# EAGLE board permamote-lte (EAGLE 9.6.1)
REV: C
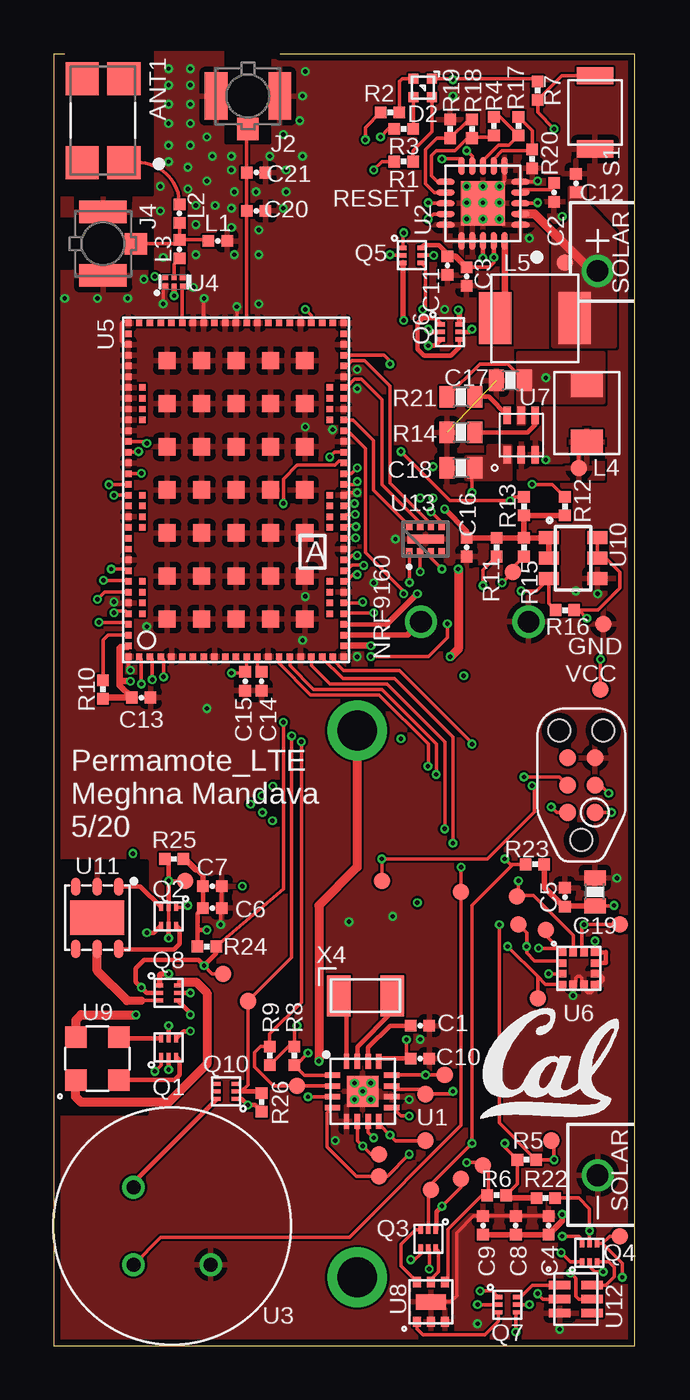
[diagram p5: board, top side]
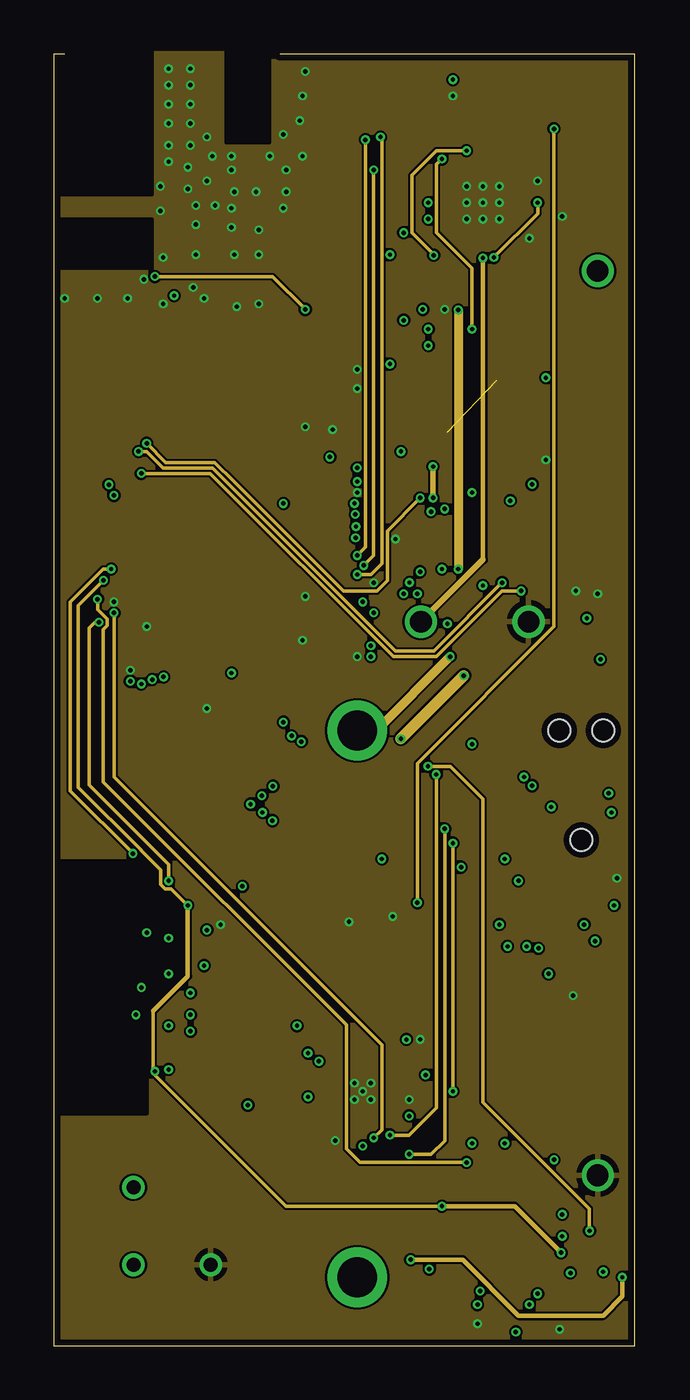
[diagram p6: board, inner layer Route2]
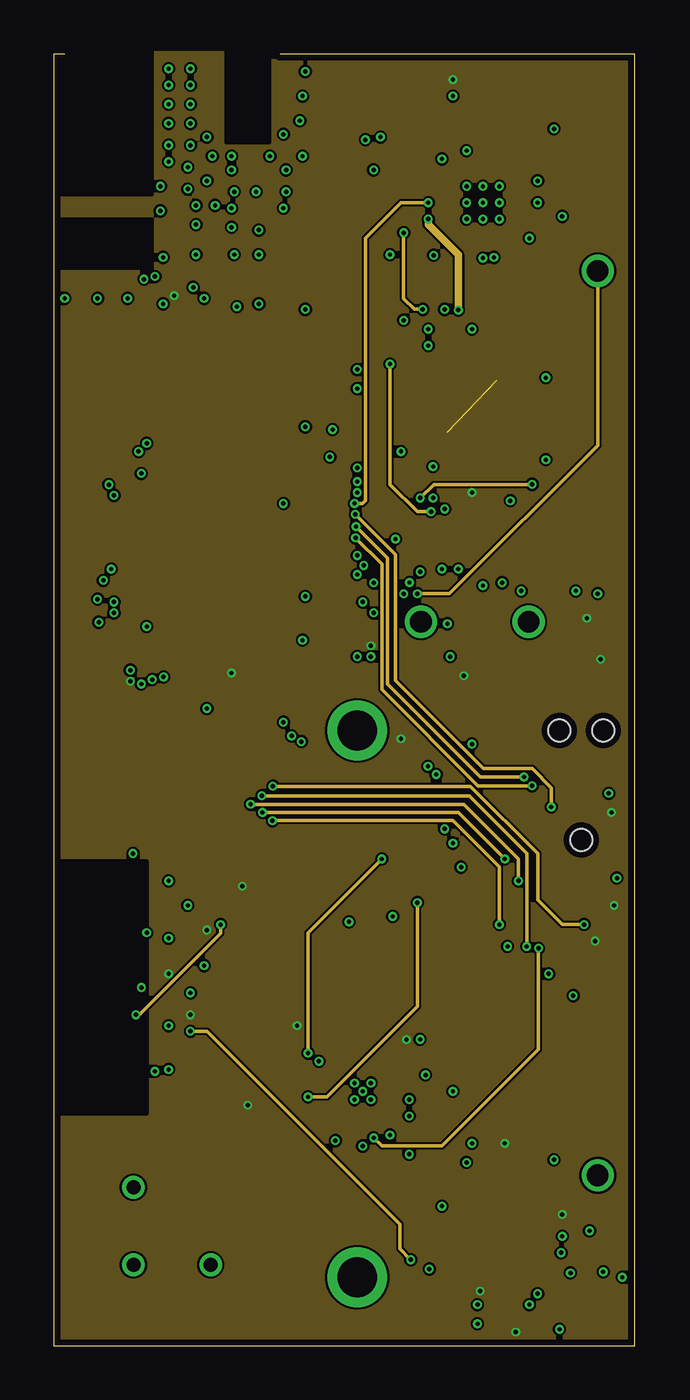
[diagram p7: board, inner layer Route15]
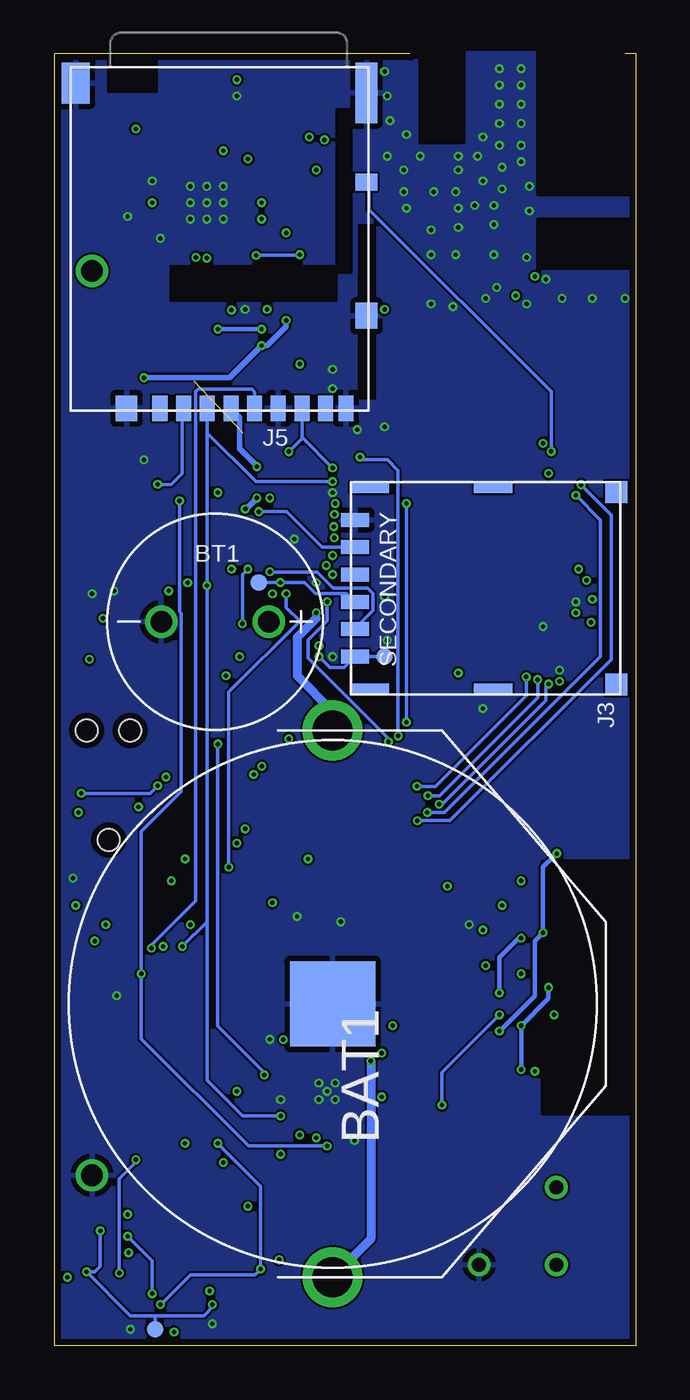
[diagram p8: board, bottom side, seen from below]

Size 27 x 60 mm. Coordinates in mm from the lower left corner, seen from the top.
Outline: 0.5,60 0,60 0,0 27,0 27,60 10.5,60
Copper layers (1+2*15+16): Top 0.0178mm / dielectric 59mil / Route2 0.0356mm / dielectric 0.1499mm / Route15 0.0356mm / dielectric 0.2007mm / Bottom 0.0178mm
Design rules "quickturn_co_kr_1oz_4lyr *": minimum track width 4mil, minimum drill 8mil, track to track 4mil, track to pad 4mil, pad to pad 4mil, via to via 4mil, smd to smd 4mil, copper to edge 12mil, drill to drill 12mil, minimum pad ring 8mil, minimum via ring 4mil, stop-mask expansion 3mil, vias tented up to drill 50mil, thermal gap 10mil
tKeepout: area 24.9,18 to 25.4,18
tRestrict: area 24.4,16.5 to 24.4,17; area 24.9,16.5 to 24.9,17; area 24.9,17 to 25.4,17; area 17.8,0.9 to 17.9,1.5

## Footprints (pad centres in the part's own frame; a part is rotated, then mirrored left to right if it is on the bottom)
ANT_1462350001 = smd 1.54 x 1.54: 1 -1.95,-0.97; 2 1.95,-0.97; 3 1.95,0.97; 4 -1.95,0.97
2477THMCOINCLIP = drill 1.854: 1 -12.7,0; 2 12.7,0 | smd 3.962 x 3.962: GND 0,0
1020 = drill 1: + -2.5,0; - 2.5,0
0402_CAP = smd 0.536 x 0.546: 1 -0.433,0; 2 0.433,0
0603_CAP = smd 0.7 x 1: 1 -0.65,0; 2 0.65,0
SOLAR_HOLES = drill 1: + 0,0; - 42,0
1MM_SQ_4PAD = smd 0.457 x 0.457: 1 0.432,0.432; 2 0.432,-0.432; 3 -0.432,-0.432; 4 -0.432,0.432
TC2030-IDC-NL = smd 0.787 x 0.787: 1 -1.27,-0.635; 2 -1.27,0.635; 3 0,-0.635; 4 0,0.635; 5 1.27,-0.635; 6 1.27,0.635 | hole 1.016: -2.54,0; 2.54,1.016; 2.54,-1.016
U.FL_SMT = smd 1.05 x 2.2: GND1 -1.475,0; GND2 1.475,0 | smd 1 x 1.05: SIG 0,-1.525
WURTH_NANO_SIM = smd 0.65 x 1.3: C1 1.905,6.07; C2 -0.635,6.07; C3 -1.905,6.07; C5 3.175,6.07; C6 0.635,6.07; C7 -3.175,6.07 | smd 1.03 x 1: P$8 -4.465,-6.07; P$9 4.465,-6.07 | smd 0.48 x 1.8: P$10 -4.66,-0.35; P$11 4.66,-0.35; P$12 -4.66,5.4; P$13 4.66,5.4
DM3AT-SF-PEJM5 = smd 0.7 x 1.2: 1 3.2,-0.1; 2 2.1,-0.1; 3 1,-0.1; 4 -0.1,-0.1; 5 -1.2,-0.1; 6 -2.3,-0.1; 7 -3.4,-0.1; 8 -4.5,-0.1; B -5.45,-0.1 | smd 1 x 0.8: A -6.4,-10.6 | smd 1 x 1.2: MOUNT0 4.75,-0.1; MOUNT1 -6.4,-4.4 | smd 1 x 2.8: MOUNT2 -6.4,-14.75 | smd 1.3 x 1.9: MOUNT3 7.1,-15.2
IHL-1212BZ-11 = smd 1.2 x 1.5: P$1 -1.35,0; P$2 1.35,0
74437324220 = smd 1.5 x 2.4: P$1 1.85,0; P$2 -1.85,0
XDFN-6 = smd 0.35 x 0.2: 1 -0.425,0.35; 2 -0.425,0; 3 -0.425,-0.35; 4 0.425,-0.35; 5 0.425,0; 6 0.425,0.35
0402_RES = smd 0.536 x 0.546: 1 -0.433,0; 2 0.433,0
0603-RES = smd 0.7 x 1: 1 -0.65,0; 2 0.65,0
B3U-1000P = smd 0.8 x 1.7: 1 -1.7,0; 2 1.7,0
PAD.03X.03 = smd 0.762 x 0.762: P$1 0,0
QFN-16-3MM = smd 0.7 x 0.25: 1 -1.4,0.75; 2 -1.4,0.25; 3 -1.4,-0.25; 4 -1.4,-0.75; 9 1.35,-0.75; 10 1.35,-0.25; 11 1.35,0.25; 12 1.35,0.75 | smd 0.25 x 0.7: 5 -0.75,-1.4; 6 -0.25,-1.4; 7 0.25,-1.4; 8 0.75,-1.4; 13 0.75,1.4; 14 0.25,1.4; 15 -0.25,1.4; 16 -0.75,1.4 | smd 1.45 x 1.45: GND 0,0
S-PVQFN-N20-RGR = smd 0.28 x 0.85: 1 -1,-1.74; 2 -0.5,-1.74; 3 0,-1.74; 4 0.5,-1.74; 5 1,-1.74; 11 1,1.74; 12 0.5,1.74; 13 0,1.74; 14 -0.5,1.74; 15 -1,1.74 | smd 0.85 x 0.28: 6 1.74,-1; 7 1.74,-0.5; 8 1.74,0; 9 1.74,0.5; 10 1.74,1; 16 -1.74,1; 17 -1.74,0.5; 18 -1.74,0; 19 -1.74,-0.5; 20 -1.74,-1 | smd 2.05 x 2.05: PAD 0,0
AMN2 = drill 0.65: GND 1.796,-1.796; OUT -1.796,-1.796; VCC -1.796,1.796
LNA-TSLP-6-2-ORIG = smd 0.25 x 0.25: 1 -0.2,0.4; 2 -0.2,0; 3 -0.2,-0.4; 4 0.2,-0.4; 5 0.2,0; 6 0.2,0.4
NRF9160 = smd 0.3 x 0.3: ANT 15.75,4.75; AUX 15.75,6.25; COEX0 5.25,10.25; COEX1 5.75,10.25; COEX2 6.25,10.25; ENABLE 1.25,10.25; GND_SHIELD@1 0.25,10.25; GND_SHIELD@2 0.25,8.25; GND_SHIELD@3 0.25,6.25; GND_SHIELD@4 0.25,3.75; GND_SHIELD@5 0.25,2.25; GND_SHIELD@6 0.25,0.25; GND_SHIELD@7 3.25,0.25; GND_SHIELD@8 5.25,0.25; GND_SHIELD@9 7.75,0.25; GND_SHIELD@10 10.25,0.25; GND_SHIELD@11 11.75,0.25; GND_SHIELD@12 13.25,0.25; GND_SHIELD@13 14.75,0.25; GND_SHIELD@14 15.75,0.25; GND_SHIELD@15 15.75,2.25; GND_SHIELD@16 15.75,4.25; GND_SHIELD@17 15.75,5.25; GND_SHIELD@18 15.75,5.75; GND_SHIELD@19 15.75,6.75; GND_SHIELD@20 15.75,7.25; GND_SHIELD@21 15.75,10.25; GND_SHIELD@22 14.75,10.25; GND_SHIELD@23 14.25,10.25; GND_SHIELD@24 13.75,10.25; GND_SHIELD@25 13.25,10.25; GND_SHIELD@26 12.75,10.25; GND_SHIELD@27 12.25,10.25; GND_SHIELD@28 11.75,10.25; GND_SHIELD@29 11.25,10.25; GND_SHIELD@30 10.75,10.25; GND_SHIELD@31 9.25,10.25; GND_SHIELD@32 6.75,10.25; GND_SHIELD@33 4.75,10.25; GND_SHIELD@34 2.75,10.25; GPS 15.75,7.75; IO_SUPPLY 0.25,4.25; MAGPIO0 15.75,1.75; MAGPIO1 15.75,1.25; MAGPIO2 15.75,0.75; NC1 0.25,7.75; NC2 0.25,7.25; NC3 0.25,6.75; NC4 0.25,5.75; NC5 0.25,5.25; NC6 15.25,0.25; NC7 15.75,8.25; NC8 15.75,8.75; NC9 15.75,9.25; NC10 15.75,9.75; NC11 15.25,10.25; NC12 2.25,0.9; NC13 2.75,0.9; NC14 3.25,0.9; NC15 3.75,0.9; NC16 6.25,0.9; NC17 6.75,0.9; NC18 7.25,0.9; NC19 7.75,0.9; NC20 11.25,0.9; NC21 11.75,0.9; NC22 12.25,0.9; NC23 12.75,0.9; NC24 12.75,9.6; NC25 12.25,9.6; NC26 11.75,9.6; NC27 11.25,9.6; NC28 7.75,9.6; NC29 7.25,9.6; NC30 6.75,9.6; NC31 6.25,9.6; NC32 3.75,9.6; NC33 3.25,9.6; NC34 2.75,9.6; NC35 2.25,9.6; NRESET 5.75,0.25; P0.00 4.25,10.25; P0.01 3.75,10.25; P0.02 3.25,10.25; P0.03 2.25,10.25; P0.04 1.75,10.25; P0.05 0.25,9.75; P0.06 0.25,9.25; P0.07 0.25,8.75; P0.08 0.25,3.25; P0.09 0.25,2.75; P0.10 0.25,1.75; P0.11 0.25,1.25; P0.12 0.25,0.75; P0.13 1.25,0.25; P0.14 1.75,0.25; P0.15 2.25,0.25; P0.16 2.75,0.25; P0.17 3.75,0.25; P0.18 4.25,0.25; P0.19 4.75,0.25; P0.20 7.25,0.25; P0.21 8.25,0.25; P0.22 8.75,0.25; P0.23 9.25,0.25; P0.24 9.75,0.25; P0.25 10.75,0.25; P0.26 10.25,10.25; P0.27 9.75,10.25; P0.28 8.75,10.25; P0.29 8.25,10.25; P0.30 7.75,10.25; P0.31 7.25,10.25; SCLK 15.75,3.25; SDATA 15.75,3.75; SIM_1V8 14.25,0.25; SIM_CLK 12.75,0.25; SIM_DET 12.25,0.25; SIM_IO 13.75,0.25; SIM_RST 11.25,0.25; SWDCLK 6.25,0.25; SWDIO 6.75,0.25; VDD@1 0.75,0.25; VDD@2 0.75,10.25; VDD_GPIO 0.25,4.75; VIO 15.75,2.75 | smd 0.8 x 0.8: GND@1 2,8.45; GND@2 4,8.45; GND@3 6,8.45; GND@4 8,8.45; GND@5 10,8.45; GND@6 12,8.45; GND@7 14,8.45; GND@8 2,6.85; GND@9 4,6.85; GND@10 6,6.85; GND@11 8,6.85; GND@12 10,6.85; GND@13 12,6.85; GND@14 14,6.85; GND@15 2,5.25; GND@16 4,5.25; GND@17 6,5.25; GND@18 8,5.25; GND@19 10,5.25; GND@20 12,5.25; GND@21 14,5.25; GND@22 2,3.65; GND@23 4,3.65; GND@24 6,3.65; GND@25 8,3.65; GND@26 10,3.65; GND@27 12,3.65; GND@28 14,3.65; GND@29 2,2.05; GND@30 4,2.05; GND@31 6,2.05; GND@32 8,2.05; GND@33 10,2.05; GND@34 12,2.05; GND@35 14,2.05
LGA-12 = smd 0.375 x 0.35: 1 -0.75,0.75; 2 -0.75,0.25; 3 -0.75,-0.25; 4 -0.75,-0.75; 7 0.75,-0.75; 8 0.75,-0.25; 9 0.75,0.25; 10 0.75,0.75 | smd 0.35 x 0.375: 5 -0.25,-0.75; 6 0.25,-0.75; 11 0.25,0.75; 12 -0.25,0.75
UDFN-6-MAXIM = smd 0.8 x 0.35: 1 -0.915,0.65; 2 -0.915,0; 3 -0.915,-0.65; 4 0.915,-0.65; 5 0.915,0; 6 0.915,0.65
UDFN-6-EXPOSED = smd 0.48 x 0.36: 1 -0.925,0.65; 2 -0.925,0; 3 -0.925,-0.65; 4 0.925,-0.65; 5 0.925,0; 6 0.925,0.65 | smd 0.71 x 1.4: EP 0,0
4-SMD = smd 1 x 1: 1 -1,1; 2 -1,-1; 3 1,-1; 4 1,1
TSOT23-6 = smd 0.6 x 0.927: 1 -0.95,-1.126; 2 0,-1.126; 3 0.95,-1.126; 4 0.95,1.126; 5 0,1.126; 6 -0.95,1.126
DFN-6/3MM = smd 0.85 x 0.45: 1 -1.45,1; 2 -1.45,0; 3 -1.45,-1; 4 1.45,-1; 5 1.45,0; 6 1.45,1 | smd 1.6 x 2.5: P$1 0,0
FN-6 = smd 1 x 0.4: 1 -0.75,0.65; 2 -0.75,0; 3 -0.75,-0.65; 4 0.75,-0.65; 5 0.75,0; 6 0.75,0.65
DPV8_1P7X0P4 = smd 0.38 x 0.3: 1 -0.61,0.75; 2 -0.61,0.25; 3 -0.61,-0.25; 4 -0.61,-0.75; 5 0.61,-0.75; 6 0.61,-0.25; 7 0.61,0.25; 8 0.61,0.75 | smd 0.4 x 1.7: 9 0,0
2-SMD = smd 1.092 x 1.905: 1 -1.245,0; 2 1.245,0

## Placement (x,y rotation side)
ANT1  1462350001  [ANT_1462350001]  2.29,56.9 90 top
BAT1  2477THMCOINCELLCLIP  [2477THMCOINCLIP]  14.1,15.88 90 bottom
BT1  LTOHTC1020  [1020]  19.56,33.62 180 bottom
C1  47pF  [0402_CAP]  17.02,14.86 0 top
C2  10nF  [0402_CAP]  23.24,53.56 270 top
C3  10nF  [0402_CAP]  19.18,49.66 270 top
C4  0.1uF  [0402_CAP]  22.99,5.59 90 top
C5  0.1uF  [0402_CAP]  23.75,20.83 90 top
C6  0.1uF  [0402_CAP]  7.37,20.32 0 top
C7  0.1uF  [0402_CAP]  7.37,21.34 0 top
C8  1uF  [0402_CAP]  21.46,5.59 90 top
C9  1uF  [0402_CAP]  19.94,5.59 90 top
C10  1uF  [0402_CAP]  17.02,13.34 0 top
C11  4.7uF  [0402_CAP]  18.29,50.16 270 top
C12  4.7uF  [0402_CAP]  24.26,53.99 90 top
C13  4.7uF  [0402_CAP]  4.06,30.1 0 top
C14  4.7uF  [0402_CAP]  9.65,30.86 270 top
C15  4.7uF  [0402_CAP]  8.89,30.86 270 top
C16  4.7uF  [0402_CAP]  19.18,37.08 270 top
C17  10uF  [0603_CAP]  21.21,44.83 180 top
C18  10uF  [0603_CAP]  18.92,40.77 180 top
C19  10uF  [0603_CAP]  25.15,21.08 90 top
C20  DNP  [0402_CAP]  9.4,52.7 180 top
C21  DNP  [0402_CAP]  9.4,54.48 180 top
D1  SOLARCELLHOLES  [SOLAR_HOLES]  25.27,49.91 270 top
D2  SML-LX0404SIUPGUSB  [1MM_SQ_4PAD]  17.14,58.42 0 top
J1  TC2030-JLINK-NL  [TC2030-IDC-NL]  24.51,26.04 90 top
J2  U.FL-R-SMT  [U.FL_SMT]  9.02,58.04 0 top
J3  NANO_SIM  [WURTH_NANO_SIM]  6.99,35.18 90 bottom
J4  U.FL-R-SMT  [U.FL_SMT]  2.29,51.18 90 top
J5  DM3AT-SF-PEJM5  [DM3AT-SF-PEJM5]  18.92,43.43 180 bottom
L1  1.8nH  [0402_CAP]  7.62,51.31 180 top
L2  5.1nH  [0402_CAP]  5.84,52.58 90 top
L3  7.5nH  [0402_CAP]  5.84,50.93 90 top
L4  1uH  [IHL-1212BZ-11]  24.77,43.31 270 top
L5  22uH  [74437324220]  22.35,47.72 180 top
Q1  PMDXB950UPEL  [XDFN-6]  5.33,13.84 90 top
Q2  PMDXB950UPEL  [XDFN-6]  5.33,19.94 270 top
Q3  PMDXB950UPEL  [XDFN-6]  17.4,4.95 270 top
Q4  PMDXB950UPEL  [XDFN-6]  24.89,4.32 90 top
Q5  PMDXB950UPEL  [XDFN-6]  16.64,50.64 0 top
Q6  PMDXB950UPEL  [XDFN-6]  18.41,47.09 0 top
Q7  PMDXB950UPEL  [XDFN-6]  21.08,1.91 0 top
Q8  PMDXB950UPEL  [XDFN-6]  5.33,16.38 0 top
Q10  PMDXB950UPEL  [XDFN-6]  8,11.81 180 top
R1  470  [0402_RES]  16.26,54.99 180 top
R2  470  [0402_RES]  15.62,57.28 180 top
R3  470  [0402_RES]  16.26,56.52 180 top
R4  6.04k  [0402_RES]  20.45,56.64 90 top
R5  10k  [0402_RES]  21.97,8.64 180 top
R6  10k  [0402_RES]  20.57,6.99 0 top
R7  10k  [0402_RES]  22.48,58.29 90 top
R8  10k  [0402_RES]  11.18,13.46 90 top
R9  10k  [0402_RES]  10.03,13.46 270 top
R10  10k  [0402_RES]  2.29,30.48 90 top
R11  10k  [0402_RES]  20.57,37.08 90 top
R12  10k  [0402_RES]  23.75,38.99 270 top
R13  10k  [0402_RES]  21.84,38.99 270 top
R14  80.6k  [0603-RES]  18.92,42.42 0 top
R15  100k  [0402_RES]  21.84,37.08 90 top
R16  100k  [0402_RES]  23.75,34.16 0 top
R17  3.9M  [0402_RES]  21.59,56.64 270 top
R18  6.2M  [0402_RES]  19.43,56.52 270 top
R19  6.8M  [0402_RES]  18.41,56.52 270 top
R20  9.1M  [0402_RES]  22.23,55.12 90 top
R21  33M  [0603-RES]  18.92,44.07 180 top
R22  100M  [0402_RES]  22.86,6.86 180 top
R23  100M  [0402_RES]  22.35,22.35 0 top
R24  100M  [0402_RES]  7.11,18.54 180 top
R25  100M  [0402_RES]  5.59,22.61 0 top
R26  100M  [0402_RES]  9.65,11.3 270 top
S1  B3U-1000P  [B3U-1000P]  25.15,57.28 90 top
TP1  TEST-POINT  [PAD.03X.03]  26.29,5.08 0 top
TP2  TEST-POINT  [PAD.03X.03]  18.92,7.75 0 top
TP3  TEST-POINT  [PAD.03X.03]  22.86,19.3 270 top
TP4  TEST-POINT  [PAD.03X.03]  15.11,8.89 0 top
TP5  TEST-POINT  [PAD.03X.03]  22.48,16.13 90 top
TP6  TEST-POINT  [PAD.03X.03]  18.16,12.57 0 top
TP7  TEST-POINT  [PAD.03X.03]  21.59,19.56 90 top
TP8  TEST-POINT  [PAD.03X.03]  7.87,17.27 0 top
TP9  TEST-POINT  [PAD.03X.03]  22.35,0.76 0 bottom
TP10  TEST-POINT  [PAD.03X.03]  17.53,7.24 0 top
TP11  TEST-POINT  [PAD.03X.03]  9.02,16 0 top
TP12  TEST-POINT  [PAD.03X.03]  6.1,21.59 0 top
TP13  TEST-POINT  [PAD.03X.03]  17.27,11.68 90 top
TP14  TEST-POINT  [PAD.03X.03]  15.11,7.87 0 top
TP15  TEST-POINT  [PAD.03X.03]  17.27,9.53 0 top
TP16  TEST-POINT  [PAD.03X.03]  11.3,12.06 0 top
TP17  TEST-POINT  [PAD.03X.03]  15.24,21.59 0 top
TP18  TEST-POINT  [PAD.03X.03]  21.51,20.87 0 top
TP19  TEST-POINT  [PAD.03X.03]  26.29,19.56 270 top
TP20  TEST-POINT  [PAD.03X.03]  23.11,9.53 0 top
TP21  TEST-POINT  [PAD.03X.03]  19.94,8.38 0 top
TP22  TEST-POINT  [PAD.03X.03]  18.92,21.08 90 top
TP23  TEST-POINT  [PAD.03X.03]  23.75,50.29 0 top
TP25  TEST-POINT  [PAD.03X.03]  24.38,40.77 0 top
TP26  TEST-POINT  [PAD.03X.03]  25.4,30.48 0 top
TP27  TEST-POINT  [PAD.03X.03]  25.53,33.53 0 top
TP30  TEST-POINT  [PAD.03X.03]  17.53,35.43 0 bottom
TP31  TEST-POINT  [PAD.03X.03]  11.68,32 270 bottom
TP32  TEST-POINT  [PAD.03X.03]  21.34,35.94 0 top
U1  AB1815-T3  [QFN-16-3MM]  14.35,11.81 0 top
U2  BQ25505  [S-PVQFN-N20-RGR]  19.94,53.05 90 top
U3  EKMB1101111  [AMN2]  5.5,5.56 0 top
U4  BGA725L6  [LNA-TSLP-6-2-ORIG]  5.59,49.4 90 top
U5  NRF9160  [NRF9160]  13.72,31.75 90 top
U6  LIS2DW12  [LGA-12]  24.38,17.53 0 top
U7  MAX17222  [UDFN-6-MAXIM]  21.72,42.29 90 top
U8  MAX44009  [UDFN-6-EXPOSED]  17.53,2.03 90 top
U9  MS5637-02BA03  [4-SMD]  2.03,13.34 90 top
U10  SIP32510  [TSOT23-6]  24.13,36.58 270 top
U11  SI7021-A20-GM1  [DFN-6/3MM]  2.02,19.88 270 top
U12  TCS34725  [FN-6]  24.26,2.16 0 top
U13  TPD3F303DPVR  [DPV8_1P7X0P4]  17.27,37.47 90 top
U$2  [UCB_CAL_200MIL]  19.81,10.54 0 top
X4  ABS07-32.768KHZ-7-T  [2-SMD]  14.48,16.26 0 top

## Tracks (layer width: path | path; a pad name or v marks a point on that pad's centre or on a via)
!CLR_EN  (via drill 0.2)
  Top 0.152: Q7.2 v19.68,1.91 | v25.53,3.43 25.15,3.43 24.89,3.68 Q4.2 | Q4.5 v24.89,5.33 24.89,6.35 24.38,6.86 R22.1 | U5.P0.08 10.47,31.7 11.94,30.23 15.11,30.23 17.4,27.94 17.4,26.92 v17.38,26.91
  Route2 0.152: v17.38,26.91 18.43,26.91 19.94,25.4 19.94,11.3 24.89,6.35 v24.89,5.33
  Bottom 0.152: v19.68,1.91 19.62,1.84 20.07,1.4 22.35,1.4 | v24.89,5.33 24.89,3.68 25.15,3.43 v25.53,3.43 23.5,1.4 22.35,1.4 | 22.35,1.4 TP9.P$1
!CLR_INT  (via drill 0.2)
  Top 0.152: U12.5 24.38,2.16 24.26,2.29 24.26,3.12 v24,3.38 | U5.P0.29 v2.56,40 v2.56,39.99 | TP20.P$1 23.24,9.4 v23.24,8.64 R5.1 20.7,10.34 v20.7,19.56
  Route15 0.152: v20.7,19.56 20.7,22.23 18.54,24.38 v10.16,24.38
  Bottom 0.152: v23.24,8.64 23.24,8.51 24,7.75 v24,3.38 | v2.56,39.99 1.14,38.58 1.14,31.88 8.64,24.38 v10.16,24.38
!HUM_EN  (via drill 0.2)
  Top 0.152: v2.09,33.59 3.37,33.59 U5.P0.04 | TP12.P$1 v5.33,21.59 | Q2.2 Q2.5
  Top 0.203: Q2.5 v5.33,18.92 | Q8.5 v6.35,16.38 | Q2.2 v5.33,21.59 5.33,22.43 R25.1
  Route2 0.152: v2.09,33.59 1.91,33.59 1.65,33.34 1.65,26.04 5.33,22.35 v5.33,21.59
  Bottom 0.203: v5.33,18.92 5.33,19.05 6.35,18.03 v6.35,16.38
!LT_EN  (via drill 0.2)
  Top 0.152: Q3.5 17.44,4.48 v17.44,3.56 | Q7.5 v22.1,1.91 | Q3.2 17.4,7.11 TP10.P$1 17.53,7.49 v19.43,9.4 19.43,20.45 21.34,22.35 | R23.1 21.34,22.35 | 21.34,22.35 21.21,22.35 v20.95,22.61 | U5.P0.30 v2.79,39.5
  Route15 0.152: v20.95,22.61 18.8,24.77 v9.7,24.77
  Bottom 0.152: v19.43,9.4 17.44,7.41 v17.44,3.56 17.7,3.3 20.7,3.3 v22.1,1.91 | v2.79,39.5 1.65,38.35 1.65,32 8.89,24.77 v9.7,24.77
!LT_INT  (via drill 0.2)
  Top 0.152: U8.4 18.3,3.08 18.3,5.4 19.89,6.99 R6.1 20.19,7.04 20.19,8.13 TP21.P$1 19.81,8.51 v19.18,8.51 | U5.P0.02 2.36,35 v2.03,34.67
  Route2 0.152: v2.03,34.67 2.03,34.19 2.47,33.75 2.47,33.44 2.29,33.25 2.29,26.19 13.59,14.89 13.59,9.14 14.22,8.51 v19.18,8.51
!PIR_EN  (via drill 0.2)
  Top 0.152: U5.P0.24 13.05,41.5 v12.83,41.27 | v11.05,28.32 11.05,18.03 TP11.P$1 9.02,12.12 8.71,11.81 Q10.2
  Top 0.203: Q10.2 9.58,11.81 R26.1
  Bottom 0.152: v11.05,28.32 11.05,40.64 11.56,41.15 12.7,41.15 v12.83,41.27
!PR_EN  (via drill 0.2)
  Top 0.152: v6.99,17.65 7.37,17.27 TP8.P$1 | R24.1 10.67,21.22 v10.67,28.96 | U5.P0.23 13.38,41.08 13.24,41.08 13.05,40.89 11.3,40.89 10.67,40.26 v10.67,39.12
  Top 0.203: Q1.5 v5.33,14.86 | Q1.2 v5.33,12.83 | Q8.2 4.32,16.38 v4.06,16.64 3.81,16.89 3.81,17.53 4.19,17.91 6.73,17.91 v6.99,17.65 7.54,18.21 R24.1
  Bottom 0.152: v10.67,39.12 v10.67,28.96
  Bottom 0.203: v5.33,12.83 v5.33,14.86 4.06,16.13 v4.06,16.64
!RST  (via drill 0.2)
  Top 0.152: U1.1 11.64,12.56 R8.1 11.25,13.03 v11.81,13.59 | U5.NRESET 13.48,37.52 v14.02,37.52 | TP17.P$1 v15.24,22.61 20.15,22.61 22.33,24.79 22.33,25.9 v22.23,26 | v25.78,25.65 25.4,26.04 J1.3
  Route15 0.152: v14.02,37.52 15.24,36.3 15.24,30.48 19.72,26 v22.23,26 | v15.24,22.61 11.81,19.18 v11.81,13.59
  Bottom 0.152: v22.23,26 22.57,25.65 v25.78,25.65
!RTC_EXTR  (via drill 0.2)
  Top 0.152: v23.24,56.52 22.48,57.28 R7.1 23.6,58.98 S1.2 | U1.3 v11.81,11.56
  Route2 0.152: v23.24,56.52 23.24,33.4 16.89,27.05 v16.89,20.57
  Route15 0.152: v16.89,20.57 16.89,15.75 12.7,11.56 v11.81,11.56
!RTC_IRQ1  (via drill 0.2)
  Top 0.152: U1.11 15.85,11.91 17.04,11.91 TP13.P$1 18.41,11.68 v18.54,11.81 | U5.P0.11 12.47,31.95 13.43,30.99 15.83,30.99 18.54,28.28 v18.54,23.34
  Route2 0.152: v18.54,23.34 v18.54,11.81
!RTC_IRQ2  (via drill 0.2)
  Top 0.152: U5.P0.10 11.97,31.59 12.83,30.73 15.47,30.73 18.16,28.05 v18.16,24 | U1.4 12.7,10.81 12.7,9.24 14.07,7.87 TP14.P$1 15.49,7.87 v16.51,8.89
  Route2 0.152: v18.16,24 18.16,9.53 17.53,8.89 v16.51,8.89
!RTC_IRQ3  (via drill 0.2)
  Top 0.152: U1.8 15.1,10.3 v15.62,9.78 15.88,9.53 TP15.P$1 | v17.77,26.53 17.78,26.54 17.78,27.94 15.24,30.48 12.06,30.48 10.97,31.58 U5.P0.09
  Route2 0.152: v17.77,26.53 17.78,26.53 17.78,11.05 16.51,9.78 v15.62,9.78
!SD_CS  (via drill 0.2)
  Top 0.152: v4.32,41.91 4.23,42 U5.P0.26 | v22.23,40.01 23.17,40.01 R12.1
  Route2 0.152: v4.32,41.91 5.21,41.02 7.48,41.02 8.37,40.13 8.38,40.13 13.46,35.05 15.02,35.05 15.49,35.53 15.49,37.85 v17.02,39.37
  Route15 0.152: v17.02,39.37 17.65,40.01 v22.23,40.01
  Bottom 0.152: J5.2 21.08,43.48 21.08,40.51 21.59,40.01 v22.23,40.01
!SD_DETECT  (via drill 0.2)
  Top 0.152: v3.94,41.53 3.91,41.5 U5.P0.27 | v20.83,35.43 v20.83,35.44 TP32.P$1 21.34,36.14 R15.1
  Route2 0.152: v3.94,41.53 4.32,41.53 5.08,40.77 7.38,40.77 15.88,32.26 17.65,32.26 v20.83,35.43
  Bottom 0.152: J5.A 12.4,53.91 12.4,52.76 3.94,44.3 v3.94,41.53
!VBAT_PRI_ON  (via drill 0.2)
  Top 0.152: v18.03,55.12 18.94,55.12 U2.10
  Top 0.203: Q6.2 17.53,47.09 v17.4,47.21 | v19.43,47.21 19.3,47.09 Q6.5
  Route2 0.152: v19.43,47.21 19.43,50.04 17.78,51.69 17.78,54.86 v18.03,55.12
  Bottom 0.203: v17.4,47.21 v19.43,47.21
!VBAT_SEC_ON  (via drill 0.2)
  Top 0.152: Q5.5 v17.65,50.64 | v19.18,55.5 19.44,55.24 U2.9 | v15.62,50.67 15.65,50.64 Q5.2
  Route2 0.152: v19.18,55.5 17.78,55.5 16.64,54.36 16.64,51.69 17.65,50.67 v17.65,50.64
  Bottom 0.152: v17.65,50.64 15.65,50.64 v15.62,50.67
ACC_CS  (via drill 0.2)
  Top 0.152: U6.2 23.54,17.87 22.34,17.87 21.97,18.24 v21.97,18.54 21.97,19.18 TP7.P$1 | U5.P0.06 4.57,31.89 v4.57,30.93
  Route15 0.152: v21.97,18.54 21.97,22.86 19.3,25.53 9.67,25.53 v9.67,25.54
  Bottom 0.152: v4.57,30.93 4.57,30.1 9.13,25.54 v9.67,25.54
ACC_INT1  (via drill 0.2)
  Top 0.152: U6.12 24.13,19.05 22.28,20.9 21.54,20.9 TP18.P$1 21.59,20.95 v21.59,21.59 | U5.P0.05 4.06,31.9 v4.06,30.73
  Route15 0.152: v9.14,25.15 19.05,25.15 21.59,22.61 v21.59,21.59
  Bottom 0.152: v4.06,30.73 4.19,30.61 4.19,29.97 9.02,25.15 v9.14,25.15
ACC_INT2  (via drill 0.2)
  Top 0.152: U6.11 24.54,18.37 24.54,19.46 v24.64,19.56 TP19.P$1 | U5.P0.07 5.1,31.87 v5.1,31.06
  Route15 0.152: v10.18,25.98 19.36,25.98 22.48,22.86 22.48,20.7 23.62,19.56 v24.64,19.56
  Bottom 0.152: v5.1,31.06 5.1,30.21 9.32,25.98 v10.18,25.98
GND  (via drill 0.2)  (1 unrouted)
  Top 0.152: v3.56,31.37 3.47,31.46 U5.GND_SHIELD@1 | U8.EP 18.43,2.03 18.73,2.33 18.73,5.24 19.5,6.02 C9.2 C8.2 C4.2 | v24.13,16.26 U6.5 | U6.5 24.24,16.89 24.24,17.07 24.32,17.14 24.45,17.14 24.52,17.07 24.52,16.89 U6.6 24.74,16.67 24.74,16.46 24.81,16.38 24.95,16.38 25.02,16.46 25.02,16.66 U6.7 25.25,16.89 25.45,16.89 25.53,16.96 25.53,17.1 25.45,17.17 25.24,17.17 U6.8 | v7.75,19.56 7.75,20.27 C6.2 C7.2 | U2.6 20.94,54.09 v20.7,53.85 | U5.GND_SHIELD@21 3.38,47.58 3.24,47.58 3.14,47.48 3.14,46.65 3.29,46.5 U5.GND_SHIELD@22 | U5.GND_SHIELD@19 6.97,48.62 arc-90 v6.99,48.64 | v5.08,48.39 5.08,49.09 U4.1 | U5.GND_SHIELD@9 13.59,39.62 v14.1,39.62 | v8.51,48.26 8.51,47.54 U5.GND_SHIELD@17 | v22.48,54.1 22.43,54.05 U2.5
  Top 0.254: U6.8 | U6.5
  Top 0.406: U9.4 1.03,15.13 1.27,15.37 v3.81,15.37
  Route15 0.152: v7.75,19.56 7.75,19.15 3.97,15.37 v3.81,15.37
  other vias: 19.18,53.85 19.94,53.85 20.7,53.09 19.94,53.09 19.18,53.09 19.18,52.32 19.94,52.32 20.7,52.32 14.35,11.81 13.97,12.19 14.73,12.19 14.73,11.43 13.97,11.43 2.03,48.64 6.48,49.15 22.86,41.15 16.51,11.43 17.02,14.22 19.68,1.02 23.5,0.76 26.16,21.72 4.32,33.4 11.68,34.8 7.11,29.59 2.79,34.54 14.86,35.43 14.1,45.34 11.56,32.77 14.1,32 25.27,34.92 24.26,35.05 8.38,50.67 9.53,48.39 9.53,50.67 5.08,50.55 6.6,50.67 9.4,53.59 7.49,52.96 4.19,49.53 8.26,51.94 9.53,51.82 10.67,52.83 8.26,52.83 8.38,53.59 10.79,53.59 8.26,54.61 10.79,54.61 3.43,48.64 4.95,52.7 6.6,52.07 6.6,52.96 6.22,53.72 5.33,54.99 6.22,54.74 0.51,48.64 4.95,53.85 7.11,56.13 7.37,55.24 8.26,55.24 10.03,55.24 11.56,55.24 11.68,59.18 6.35,59.31 5.33,59.31 5.33,58.55 6.35,58.55 6.35,57.66 5.33,57.66 5.33,56.77 6.35,56.77 6.35,55.75 5.33,55.75 7.11,54.1 11.56,58.04 11.43,56.9 10.67,56.26 13.08,9.53 11.68,42.67 12.95,42.55 14.1,44.45 22.1,51.44 18.16,48.13 13.72,19.68 15.75,19.94 23.62,52.45 18.54,58.04 15.88,37.47
  pour Top (rank 2): 0,60 27,60 27,0 0,0
  pour Bottom (rank 2): 0,60 27,60 27,0 0,0
  pour Route2 (rank 2): 0,60 0,0 27,0 27,60
GPS_EN  (via drill 0.2)
  Top 0.152: v4.7,49.66 4.75,49.6 U4.6 | v11.68,48.13 11.97,47.85 U5.MAGPIO0
  Route2 0.152: v4.7,49.66 10.16,49.66 v11.68,48.13
LBST
  Top 0.152: U2.20 20.95,51.3
  Top 0.305: 20.95,51.3 20.95,48.17
  Top 0.406: 20.95,48.17 L5.P$1
LED_BLUE  (via drill 0.2)
  Top 0.152: R3.2 15.56,56.52 v15.18,56.13 | v14.1,35.81 13.91,35.81 13.59,35.5 U5.P0.17
  Route2 0.152: v15.18,56.13 15.24,56.13 15.24,36.32 14.73,35.81 v14.1,35.81
LED_GREEN  (via drill 0.2)
  Top 0.152: R2.2 14.48,56.57 v14.48,56.01 | v14.1,36.7 13.84,36.7 | 13.84,36.7 | 13.84,36.7 13.64,36.5 U5.P0.19
  Route2 0.152: v14.1,36.7 14.48,37.08 v14.48,56.01
LED_RED  (via drill 0.2)
  Top 0.152: U5.P0.18 13.59,36 13.85,36.25 14.38,36.25 v14.39,36.24 | R1.2 15.24,54.99 v14.86,54.61
  Route2 0.152: v14.39,36.24 14.86,36.7 v14.86,54.61
MISO  (via drill 0.2)
  Top 0.152: U6.3 v22.99,17.27 | U5.P0.22 13.83,40.5 v14.1,40.77 | TP4.P$1 14.73,8.89 v14.35,9.27 14.1,9.52 U1.6 | v16.13,41.53 18.41,39.24 v21.21,39.24 21.39,39.42 R13.1
  Bottom 0.152: v14.1,40.77 15.52,42.19 J5.7 15.52,42.13 v16.13,41.53 | v14.35,9.27 18,9.27 22.99,14.26 v22.99,17.27 22.96,17.27 22.99,17.3 22.99,23.88 21.13,25.73 21.13,34.01 21.21,34.09 21.21,35.59 v21.21,39.24
MOSI  (via drill 0.2)
  Top 0.152: v16.51,10.67 16.13,10.67 15.74,11.06 U1.9 | v21.08,18.54 22.48,17.14 | 22.48,17.14 22.85,16.78 U6.4 | TP5.P$1 22.48,17.14 | v14.1,40.13 13.96,40 U5.P0.21 | v19.94,35.31 19.94,36.02 R11.1
  Bottom 0.152: v14.1,40.13 17.66,40.13 19.92,42.39 J5.3 19.92,35.32 v19.94,35.31 19.94,19.68 | v16.51,10.67 18.29,10.67 19.94,12.32 19.94,19.68 | 19.94,19.68 v21.08,18.54
N$1
  Top 0.152: U5.GPS 5.97,48.61 5.97,49.18 U4.3
N$2
  Top 0.152: U4.5 5.59,50.24 L3.1
N$4
  Top 0.152: L2.1 L3.2 | L3.2 5.62,51.18 J4.SIG | L3.2 7.2,51.36 L1.2
N$5
  Top 0.152: L2.2 arc90 3.91,54.95 ANT1.1
N$8
  Top 0.152: U5.ANT C20.2 C21.2 8.96,56.46 J2.SIG
N$9
  cutout Top: 0,52.32 4.57,52.32 4.57,50.16 4.57,50.04 0,50.04
N$10
  cutout Top: 0,22.48 1.78,22.48 1.78,20.95 2.29,20.95 2.29,22.48 4.32,22.48 4.32,10.79 0,10.79
  cutout Route2: 0,22.48 1.78,22.48 2.29,22.48 4.32,22.48 4.32,10.79 0,10.79
  cutout Route15: 0,22.48 1.78,22.48 2.29,22.48 4.32,22.48 4.32,10.79 0,10.79
  cutout Bottom: 0,22.48 1.78,22.48 2.29,22.48 4.32,22.48 4.32,10.79 0,10.79
N$11
  cutout Route2: 0,52.32 4.57,52.32 4.57,50.04 0,50.04
N$12
  Top 0.152: 22.37,42.78 U7.4
  Top 0.203: 22.37,42.78 22.01,42.42 R14.2
N$13  (via drill 0.2)
  Top 0.152: R15.2 21.84,37.65
  Top 0.254: U10.2 U10.1 23,37.52 R15.2 R11.2 C16.1 19.18,37.85 v18.16,38.86 | R12.2 R13.2 21.84,37.65
  Route2 0.254: v17.62,40.83 v17.62,39.37
  Bottom 0.152: 17.62,40.86 v17.62,40.83
  Bottom 0.254: J5.4 18.41,43.13 18.41,41.66 17.62,40.86 | v17.62,39.37 18.13,38.86 v18.16,38.86
N$14
  Top 0.203: U7.6 20.2,44.07 R21.1
N$15
  Top 0.152: D2.2 17.58,56.39 16.69,55.5 R1.1
N$16
  cutout Top: 4.57,59.94 0,59.94 0,53.47 4.57,53.47
N$17
  Top 0.152: D2.4 16.2,58.85 16.08,58.73 16.05,58.73 R2.1
N$18
  Top 0.152: R17.1 22.23,56.44 R20.2 22.17,55.5 20.83,55.5 20.44,55.11 U2.7
N$19
  Top 0.152: D2.3 16.71,56.54 R3.1
N$20
  Top 0.152: U8.1 16.88,0.78 17.14,0.51 20.02,0.51 20.66,1.14 Q7.3
N$21
  Top 0.203: Q8.6 5.92,16.89
  Top 0.406: 5.92,16.89 6.6,16.89 7.11,16.38 7.11,13.08 5.33,11.3 1.27,11.3 1.02,11.56 1.02,12.32 U9.1
N$22
  Top 0.152: 4.06,16.03 Q8.3
  Top 0.381: 3.4,16.03 4.06,16.03
  Top 0.406: 3.4,16.03 2.02,17.41 U11.5
N$23
  Top 0.203: Q10.6 3.7,7.58 U3.VCC
N$24
  cutout Route2: 4.57,59.94 0,59.94 0,53.47 4.57,53.47
N$25
  Top 0.203: U1.14 14.61,13.84 15.62,14.86 C1.1
N$26
  cutout Route15: 4.57,53.47 0,53.47 0,59.94 4.57,59.94
N$27
  cutout Bottom: 4.57,53.47 0,53.47 0,59.94 4.57,59.94
N$28
  Top 0.152: R10.2 2.29,32.77 2.52,33 U5.ENABLE
N$29
  Top 0.152: U5.IO_SUPPLY 9.47,31.48 C14.1
N$30
  cutout Route15: 0,52.32 4.57,52.32 4.57,50.04 0,50.04
N$31
  Top 0.152: Q7.6 21.69,2.25 22.23,2.79 23.49,2.79 U12.1
N$32
  Top 0.152: U2.8 19.94,55.03 20.66,55.75 21.13,55.75 R17.2 20.72,57.08 R4.2
N$34
  Top 0.152: Q1.6
  Top 0.203: U9.3 3.1,14.27 Q1.6
N$35
  cutout Bottom: 4.57,52.32 0,52.32 0,50.04 4.57,50.04
N$36
  cutout Bottom: 8,59.94 8,55.88 10.03,55.88 10.03,59.94
N$37
  cutout Route15: 8,59.94 10.03,59.94 10.03,55.88 8,55.88
N$38
  cutout Route2: 8,59.94 10.03,59.94 10.03,55.88 8,55.88
N$39
  cutout Top: 10.03,59.94 8,59.94 8,55.88 10.03,55.88
N$40
  Top 0.203: U1.15 14.1,13.87 15.72,15.49 X4.2
N$41
  Top 0.203: U9.2 5.08,12.34 5.6,12.34 5.84,12.57 5.84,13.26 Q1.3
N$43
  Top 0.203: X4.1 13.6,15.89 U1.16
N$45  (via drill 0.2)
  Top 0.152: v17.14,48.13 17.27,48.26 17.27,50.08 Q5.4 | v16.26,51.69 16.21,51.65 Q5.1
  Route15 0.152: v17.14,48.13 16.76,48.13 16.26,48.64 v16.26,51.69
N$48
  Top 0.152: Q2.3
  Top 0.203: U11.1 4.02,21.32 Q2.3
N$50
  Top 0.152: Q2.6
  Top 0.203: U11.6 3.03,18.41 5.59,18.41 5.84,18.67 5.84,19.36 Q2.6
N$51
  Top 0.152: U8.6 16.13,3.7 16.13,4.7 16.81,5.38 Q3.3
N$52
  Top 0.152: Q3.6 17.88,4.4 17.88,3.43 17.53,3.08 U8.5
N$53
  Top 0.152: 18.84,46.37 Q6.4
  Top 0.203: Q6.1 17.7,47.72 17.14,47.72 16.89,47.47 16.89,46.28 17.19,45.99 18.46,45.99 18.84,46.37
N$54
  Top 0.152: U12.6 25.64,2.81 26.04,3.2 26.04,3.64 25.78,3.89 Q4.3
N$55  (via drill 0.2)
  Top 0.152: v22.48,2.41 22.73,2.16 U12.2 | Q4.6 24.54,4.92 24.38,5.08 v23.62,5.08
  Bottom 0.152: v23.62,5.08 22.48,3.94 v22.48,2.41
N$57
  Top 0.152: U2.12 17.69,53.55 17.27,53.98 17.27,55.55 17.8,56.08 R19.2 19.28,56.95 R18.1
N$58
  Top 0.152: U2.11 17.83,54.05 17.54,54.34 17.54,55.26 17.78,55.5 18.64,55.5 19.22,56.08 R18.2 19.48,56.13 20.36,56.13 R4.1
PIR_OUT  (via drill 0.2)
  Top 0.152: U3.OUT 4.97,5.03 13.73,5.03 18.92,10.22 TP22.P$1 v18.92,22.23 | U5.P0.25 13.63,42.5 14.48,41.66 14.48,36.83 16.26,35.05 v16.26,34.92
  Bottom 0.152: v18.92,22.23 18.92,30.35 15.62,33.66 16.26,34.29 v16.26,34.92
RTC_CS  (via drill 0.2)
  Top 0.152: U1.12 15.71,12.57 v17.27,12.57 TP6.P$1 | U5.P0.12 12.97,31.87 13.47,31.37 16.06,31.37 19.43,28 v19.43,27.94
  Bottom 0.152: v19.43,27.94 19.43,14.86 17.27,12.7 v17.27,12.57
SCK  (via drill 0.2)
  Top 0.152: U1.7 14.6,9.91 v14.86,9.65 | v2.79,34.04 2.88,34.13 3.34,34.13 U5.P0.03 | v22.52,18.46 23.45,18.46 U6.1 22.86,19.05 TP3.P$1
  Route2 0.152: v2.79,34.04 2.79,26.42 15.24,13.97 15.24,10.03 v14.86,9.65
  Route15 0.152: v22.52,18.46 22.52,13.76 18.03,9.27 15.24,9.27 v14.86,9.65
  Bottom 0.152: J5.5 17.72,44.3 17.85,44.42 20.34,44.42 20.45,44.31 20.45,20.65 22.52,18.58 v22.52,18.46
SCL  (via drill 0.2)
  Top 0.152: v23.57,4.32 24,3.89 Q4.1 | Q2.1 6.14,20.36 v6.22,20.45 | TP2.P$1 18.92,7.37 v18.03,6.48 | U5.P0.01 3.42,35.55 v2.3,35.55 | v4.7,12.74 4.98,13.03 Q1.1
  Top 0.203: v18.03,6.48 17.78,6.22 17.78,5.41 Q3.1
  Route2 0.152: v18.03,6.48 10.79,6.48 4.62,12.65 4.62,12.66 | v2.3,35.55 1.14,34.39 1.14,25.93 4.06,23.01 4.06,22.99 4.95,22.1 4.95,21.43 5.18,21.21 5.46,21.21 v6.22,20.45 | 4.62,15.56 4.62,12.66 | 4.62,12.66 v4.7,12.74
  Route2 0.203: v23.57,4.32 21.41,6.48 v18.03,6.48 | v6.22,20.45 6.22,17.16 4.62,15.56
SD_ENABLE  (via drill 0.2)
  Top 0.152: v4.06,40.51 3.48,40.51 U5.P0.28 | R16.1 23,34.48 U10.3 22.43,35.05 v21.72,35.05
  Route2 0.152: v4.06,40.51 7.27,40.51 15.78,32 17.78,32 20.83,35.05 v21.72,35.05
SDA  (via drill 0.2)
  Top 0.152: Q3.4 17.05,4.27 16.77,3.99 v16.58,3.99 | Q4.4 25.5,4.74 | 25.5,4.74 26.42,3.82 v26.42,3.17 | v2.67,36.07 3.4,36.07 U5.P0.00 | 25.5,4.74 25.83,5.08 TP1.P$1
  Top 0.203: Q2.4 4.65,19.18 v4.32,19.18 | Q1.4 6.02,14.61 v6.35,14.61
  Route2 0.152: v3.68,22.86 0.76,25.77 0.76,34.54 2.29,36.07 v2.67,36.07
  Route2 0.203: v16.58,3.99 16.96,3.99 16.97,3.99 19,3.99 21.59,1.4 25.53,1.4 26.42,2.29 v26.42,3.17
  Route15 0.152: v6.35,14.61 7.11,14.61 16.07,5.64 16.07,4.5 v16.58,3.99
  Bottom 0.152: v3.68,22.86 3.8,22.73 3.81,22.73
  Bottom 0.203: v6.35,14.61 4.7,16.26 4.7,18.8 v4.32,19.18 4.32,22.23 3.81,22.73
SIM_1V8  (via drill 0.2)
  Top 0.152: v17.53,38.73 18.02,38.24 U13.5 | v15.62,45.59 15.62,45.72 15.33,46.01 U5.SIM_1V8
  Route15 0.152: v17.53,38.73 16.89,38.73 15.62,40.01 v15.62,45.59
  Bottom 0.152: J3.C1 14.58,37.08 16.23,38.73 v17.53,38.73
SIM_CLK
  Top 0.152: U5.SIM_CLK 13.59,44.5 13.97,44.88 14.3,44.88 15.24,43.94 15.24,40.01 17.02,38.22 U13.7
SIM_CLK2  (via drill 0.2)
  Top 0.152: v17.02,35.94 17.02,36.07 U13.2
  Bottom 0.152: v17.02,35.94 14.83,35.94 14.07,35.18 12.47,35.18 12.23,34.94 12.23,34.15 13.05,33.32 J3.C3
SIM_IO
  Top 0.152: U5.SIM_IO 13.59,45.5 13.85,45.75 14.44,45.75 15.62,44.58 15.62,40.07 17.52,38.17 U13.6
SIM_IO2  (via drill 0.2)
  Top 0.152: v18.29,33.53 18.29,32.89 17.4,32 v14.73,32 | v18.03,36.07 17.52,36.58 U13.3
  Bottom 0.152: TP31.P$1 J3.C7 13.56,31.5 14.22,31.5 v14.73,32 | v18.29,33.53 18.29,35.81 v18.03,36.07
SIM_RST
  Top 0.152: U13.8 14.86,39.74 14.86,42.04 13.9,43 U5.SIM_RST
SIM_RST2  (via drill 0.2)
  Top 0.152: v16.52,35.45 U13.1
  Bottom 0.152: TP30.P$1 16.53,35.43 v16.52,35.45 16.51,35.43 15.4,35.43 14.89,34.93 13.44,34.93 J3.C2
SW
  Top 0.152: TP25.P$1 24.38,41.58 L4.P$2
  pour Top: 21.84,41.91 21.59,41.91 21.59,40.26 25.53,40.26 25.53,42.55 24,42.55 24,41.02 23.75,40.77 22.1,40.77 21.84,41.02
SWDCLK  (via drill 0.2)
  Top 0.152: J1.4 23.5,26.42 v21.84,26.42 | U5.SWDCLK 13.57,38.1 13.98,38.1 v14.04,38.04
  Route15 0.152: v14.04,38.04 15.49,36.59 15.49,30.73 19.81,26.42 v21.84,26.42
SWDIO  (via drill 0.2)
  Top 0.152: U5.SWDIO 13.57,38.61 v14.01,38.61 | J1.2 23.37,24.77 v23.11,25.02
  Route15 0.152: v14.01,38.61 15.88,36.74 15.88,30.89 19.97,26.8 22.23,26.8 23.11,25.91 v23.11,25.02
VBAT  (via drill 0.2)
  Top 0.152: Q6.6 18.84,47.59 | U2.14 17.63,52.55 v17.4,52.32 | v14.86,34.04 13.5,34.04 U5.P0.15
  Top 0.254: v18.8,48.1 18.84,48.1 18.84,47.59
  Top 0.406: v18.8,36.07 18.8,32.35 18.45,32 v18.41,32 | BAT1.2 14.1,22.23 12.32,20.45 v12.32,13.21
  Route2 0.406: v18.8,48.1 v18.8,36.07 | BAT1.2 15.02,28.57 15.02,28.61 v18.41,32
  Route15 0.356: v17.4,52.32 17.4,52.07 18.8,50.67 v18.8,48.1
  Bottom 0.356: 14.86,33.78 v14.86,34.04
  Bottom 0.406: 14.86,33.78 15.75,32.89 15.75,31.11 14.1,29.46 BAT1.2 | BAT1.1 12.32,4.95 v12.32,13.21
VBAT_OK  (via drill 0.2)
  Top 0.152: v17.4,53.09 17.43,53.05 U2.13 | v13.97,39.12 13.95,39.13 13.73,39.13 13.59,39 U5.P0.20
  Route15 0.152: v17.4,53.09 16.13,53.09 14.48,51.44 14.48,39.24 14.35,39.12 v13.97,39.12
VCC  (via drill 0.2)
  Top 0.152: Q7.4 21.46,1.51 v21.46,0.64 | Q7.1 20.37,2.54 v19.81,2.54 | U5.VDD@2 3.42,32.45 | 2.34,30.1 R10.1 | 6.6,22.1 6.93,21.77 | 6.35,15.44 v6.35,15.37 | R7.2 22.35,58.85 18.54,58.85 | 18.54,58.85 D2.1 | v18.54,58.8 18.54,58.85 | C10.1 16.38,13.54 v16.38,14.22 | U5.VDD@1 13.48,32.51 | v25.15,18.8 25.15,18.29 U6.10 | v26.04,20.45 26.01,20.42 25.13,20.42 | v25.91,24.77 J1.1 | v19.43,39.62 19.43,40.62 C18.1 | R9.2 10.9,13.89 R8.2 11.18,14.73 v11.3,14.86 | R6.2 21.54,7.52 R5.2 20.95,9.22 v20.95,9.4 | U10.6 U10.5 25.65,36.58 26.29,35.94 26.29,35.18 25.27,34.16 R16.2 24.38,34.16 v24.77,33.78 | U5.VDD_GPIO 8.97,31.21 C15.1 8.84,31.24 v8.26,31.24 | U1.13 15.22,13.34 | TP26.P$1 v25.4,31.88
  Top 0.203: 15.22,13.34 C10.1 | C7.1 C6.1 6.68,20.07 6.68,19.3 | R24.2 6.68,19.3 | 6.68,19.3 v7.11,19.3 | 25.13,20.42 C19.1 | U6.9 25.65,17.78 25.65,18.29 25.64,18.28 U6.10 | Q8.4 6.35,15.44 | Q10.1 8.73,11.46 v9.02,11.18 9.35,11.18 R26.2
  Top 0.254: C9.1 C8.1 C4.1 23.62,5.79 v23.62,6.1 | R22.2 21.13,6.86 R6.2 | C19.1 23.79,20.43 C5.1 23.67,20.39 22.79,21.28 R23.2 | R25.2 6.1,22.61 6.6,22.1 | 6.93,21.77 C7.1 | Q8.1 4.91,17.19 4.99,17.27 v5.33,17.27 | U4.2 v5.59,48.77
  Top 0.305: 3.42,32.45 3.12,32.45 3.06,32.4 3.06,30.99 | 2.34,30.1 C13.1 3.06,30.67 3.06,30.99 | v3.56,30.86 3.19,30.86 3.06,30.99 | 13.48,32.51 v14.73,32.51
  Route2 0.508: v19.05,31.11 v16.13,28.19
  Bottom 0.152: v6.35,15.37 9.02,12.7 v9.02,11.18
  other vias: 8.76,21.34
  pour Top (isolate 0.203, no thermals): 20.19,41.78 21.21,41.78 21.21,40.26 19.18,40.26 19.18,41.27 20.19,41.27
  pour Route15 (rank 2): 0,60 27,60 27,0 0,0
VOC_SAMP_VSTOR  (via drill 0.2)
  Top 0.152: v20.45,50.55 20.45,50.29 20.25,50.09 C3.1 | v22.48,53.09 22.45,53.05 U2.3
  Top 0.203: v20.45,50.55 20.44,50.78 U2.19 | Q5.6 17.19,51.12 17.89,51.12 18.29,50.73 C11.1
  Top 0.254: C3.1 18.67,50.6 C11.1
  Route2 0.152: v22.48,53.09 22.48,52.58 v20.45,50.55
VREF_SAMP
  Top 0.152: U2.4 21.81,53.68 23.13,53.68 C2.1
VSEC  (via drill 0.2)
  Top 0.203: U2.18 v19.94,50.51
  Top 0.254: U5.P0.13 16.43,33 BT1.+
  Route2 0.203: v19.94,50.51 19.94,36.5
  Route2 0.254: 19.94,36.5 BT1.+
VSOL  (via drill 0.2)
  Top 0.203: 15.47,33.5 U5.P0.14
  Top 0.254: v16.89,34.92 15.47,33.5
  Top 0.406: U2.2 22.34,52.55 24.99,49.91 D1.+
  Route15 0.152: D1.+ 25.27,41.81 18.38,34.92 v16.89,34.92
  pour Top (no thermals): 24,53.76 24,52.29 23.24,51.53 23.24,46.45 26.04,46.45 26.04,51.66 24.64,53.05 24.64,53.76
VSW  (via drill 0.2)
  Top 0.152: C17.1 21.1,45.59 19.8,45.59 R21.2
  Top 0.203: Q6.3 17.7,46.45 v17.4,46.45
  Top 0.254: v16.26,47.62 16.21,47.67 Q5.3
  Bottom 0.254: v16.26,47.62 16.26,47.34 17.14,46.45 v17.4,46.45 18.89,44.96 v22.86,44.96
  pour Top (isolate 0.203, no thermals): 21.59,42.8 21.59,46.1 25.53,46.1 25.53,43.81 21.84,43.81 21.84,42.8
WDI  (via drill 0.2)
  Top 0.152: v14.35,34.54 14.31,34.5 U5.P0.16 | v11.5,28.05 11.5,15.95 10.03,14.48 R9.1 9.6,13.89 9.33,13.62 9.33,12.94 10.21,12.06 TP16.P$1 | TP16.P$1 U1.2 | TP16.P$1
  Bottom 0.152: v14.35,34.54 14.35,33.66 15.24,32.77 15.24,31.94 11.43,28.13 v11.5,28.05

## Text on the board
bPlace: SECONDARY
tNames: RESET | SOLAR | A | GND | VCC | Permamote_LTE / Meghna Mandava / 5/20 | SOLAR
